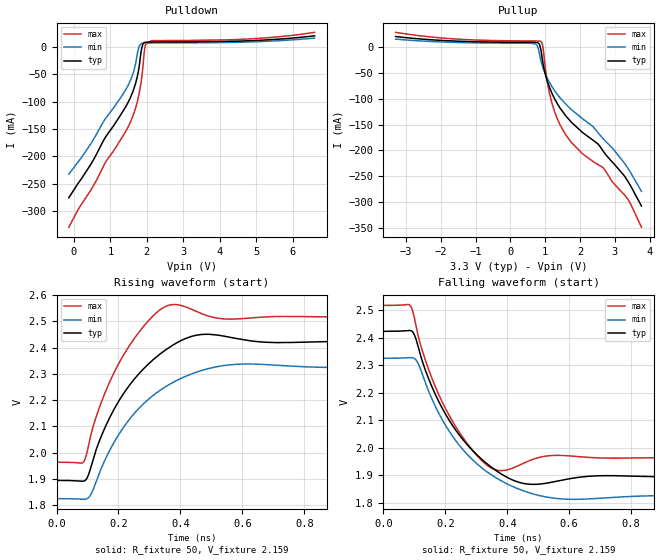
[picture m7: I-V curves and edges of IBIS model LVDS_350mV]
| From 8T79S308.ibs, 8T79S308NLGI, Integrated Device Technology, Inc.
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[Model]   LVDS_350mV
Model_type   Output
Polarity   Non-Inverting
|   typ   min   max
C_comp   2pF   1.5pF   2.5pF
Vmeas = 2.159V
Rref = 50
Cref = 0
Vref = 2.159V
|   typ   min   max
[Voltage range]   3.3V   3.135V   3.465V
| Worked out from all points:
|   slope of the pulldown table from 0 to 0.495 V, typ, clamps not added: 9.85 ohm
|   slope of the pullup table from 0 to 0.495 V, typ, clamps not added: 3.02 kohm
|   rising waveform, R_fixture 50, V_fixture 2.159: 20-80 % time 154ps typ, 180ps min, 122ps max; typ from 1.89 V to 2.42 V
|   falling waveform, R_fixture 50, V_fixture 2.159: 20-80 % time 154ps typ, 180ps min, 122ps max; typ from 2.42 V to 1.89 V
[Pulldown]
|Voltage   I (typ)   I (min)   I (max)
|Note, modeling breaks down at 250mA and above.  This is well beyond the functional   |
|operating range of the device.  Should this scenario occur, catastrophic failure and   |
|possible damage to the device and/or board is of higher concern than the I-V curve   |
|behavior.  The IBIS checker will flag currents in excess of 10A with warnings.  Lines   |
|with currents in excess of 0.35 A have been commented out.  The points still remain|
|available to the user if the user desires to use them.   |
|-1.60000e+00   -9.36050e-01   -8.30532e-01   -1.09194e+00
|-1.58360e+00   -9.23451e-01   -8.19980e-01   -1.07602e+00
|-1.51800e+00   -8.73064e-01   -7.77803e-01   -1.01237e+00
|-1.38680e+00   -7.72248e-01   -6.93503e-01   -8.84958e-01
|-1.32120e+00   -7.21791e-01   -6.51361e-01   -8.21228e-01
|-1.30480e+00   -7.09172e-01   -6.40828e-01   -8.05295e-01
|-1.27200e+00   -6.83929e-01   -6.19757e-01   -7.73430e-01
|-1.14080e+00   -5.82896e-01   -5.35437e-01   -6.46183e-01
|-1.07520e+00   -5.32359e-01   -4.93249e-01   -5.82891e-01
|-1.04240e+00   -5.07094e-01   -4.72151e-01   -5.51375e-01
|-9.76800e-01   -4.56591e-01   -4.29949e-01   -4.88499e-01
|-9.60400e-01   -4.43978e-01   -4.19400e-01   -4.73586e-01
|-9.27600e-01   -4.18775e-01   -3.98303e-01   -4.59203e-01
|-8.62000e-01   -3.73001e-01   -3.56137e-01   -4.46935e-01
|-7.96400e-01   -3.57891e-01   -3.14301e-01   -4.36605e-01
|-7.47200e-01   -3.51027e-01   -2.97867e-01   -4.28708e-01
|-6.81600e-01   -3.42516e-01   -2.88038e-01   -4.17953e-01
|-5.50400e-01   -3.25813e-01   -2.73543e-01   -3.96026e-01
|-5.34000e-01   -3.23742e-01   -2.71817e-01   -3.93266e-01
|-4.19200e-01   -3.09364e-01   -2.59932e-01   -3.73966e-01
|-4.02800e-01   -3.07325e-01   -2.58260e-01   -3.71225e-01
-140.4mV  -275.5mA   -232.5mA   -329.3mA
466.4mV   -214mA     -176.5mA   -261.2mA
860mV     -165.2mA   -131.3mA   -211.4mA
1.549V    -92.3mA    -61.1mA    -137.2mA
1.696V    -64.81mA   -28.55mA   -110.1mA
1.795V    -32.56mA   1.867mA    -82.65mA
1.877V    2.498mA    7.079mA    -45.82mA
1.926V    8.06mA     7.495mA    -10.52mA
1.959V    8.947mA    7.572mA    4.602mA
2.123V    9.35mA     7.638mA    11.84mA
4.73V     11.45mA    9.297mA    14.72mA
6.6V      20.66mA    16.55mA    27.05mA
[Pullup]
|Voltage   I (typ)   I (min)   I (max)
|Note, modeling breaks down at 250mA and above.  This is well beyond the functional   |
|operating range of the device.  Should this scenario occur, catastrophic failure and   |
|possible damage to the device and/or board is of higher concern than the I-V curve   |
|behavior.  The IBIS checker will flag currents in excess of 10A with warnings.  Lines   |
|with currents in excess of 0.35 A have been commented out.  The points still remain|
|available to the user if the user desires to use them.   |
-3.3V     20.66mA    15.57mA    28.83mA
719.4mV   9.383mA    6.524mA    12.05mA
798.6mV   8.199mA    -2.249mA   12mA
877.8mV   -5.663mA   -26.39mA   10.96mA
937.2mV   -31.68mA   -40.05mA   -604.3uA
1.016V    -55.6mA    -53.79mA   -47.49mA
1.115V    -76.39mA   -67.37mA   -86.96mA
1.432V    -118.4mA   -98.48mA   -151.1mA
2.066V    -164.9mA   -138.1mA   -206mA
2.68V     -202.6mA   -178.2mA   -234.6mA
3.373V    -259.2mA   -234.1mA   -294.4mA
3.769V    -307.8mA   -279.4mA   -348.7mA
| 3.84780e+00   -3.18622e-01   -2.89838e-01   -3.61401e-01
| 3.92700e+00   -3.29799e-01   -3.10228e-01   -3.74242e-01
| 3.96660e+00   -3.35470e-01   -3.35012e-01   -3.80702e-01
| 4.12500e+00   -3.60005e-01   -4.37435e-01   -4.06822e-01
| 4.16460e+00   -3.71679e-01   -4.63034e-01   -4.13410e-01
| 4.18440e+00   -3.83289e-01   -4.75832e-01   -4.16714e-01
| 4.22400e+00   -4.13932e-01   -5.01423e-01   -4.23349e-01
| 4.24380e+00   -4.29251e-01   -5.14216e-01   -4.26683e-01
| 4.40220e+00   -5.51718e-01   -6.16484e-01   -4.57199e-01
| 4.48140e+00   -6.12900e-01   -6.67560e-01   -5.22591e-01
| 4.50120e+00   -6.28190e-01   -6.80327e-01   -5.41875e-01
| 4.58040e+00   -6.89334e-01   -7.31378e-01   -6.18981e-01
| 4.89720e+00   -9.33601e-01   -9.36352e-01   -9.26929e-01
| 4.93680e+00   -9.64105e-01   -9.63467e-01   -9.65380e-01
| 4.95660e+00   -9.79356e-01   -9.77439e-01   -9.84604e-01
| 4.99620e+00   -1.00984e+00   -1.00618e+00   -1.02305e+00
| 5.07540e+00   -1.07073e+00   -1.06591e+00   -1.09992e+00
| 5.23380e+00   -1.19275e+00   -1.06591e+00   -1.25364e+00
| 5.31300e+00   -1.25569e+00   -1.06591e+00   -1.33049e+00
| 5.35260e+00   -1.28878e+00   -1.06591e+00   -1.36892e+00
| 5.51100e+00   -1.42874e+00   -1.06591e+00   -1.52275e+00
| 5.66940e+00   -1.42874e+00   -1.06591e+00   -1.67704e+00
| 5.76840e+00   -1.42874e+00   -1.06591e+00   -1.77893e+00
| 5.92680e+00   -1.42874e+00   -1.06591e+00   -1.95172e+00
| 5.94660e+00   -1.42874e+00   -1.06591e+00   -1.97363e+00
[Ramp]
|   typ   min   max
dV/dt_r   0.335/0.172n   0.309/0.191n   0.362/0.142n
dV/dt_f   0.335/0.172n   0.309/0.191n   0.362/0.142n
R_load =   50.0000
[Rising Waveform]
R_fixture = 50
V_fixture   =2.159  |Vcc_typ
V_fixture_min=2.075  |Vcc_min
V_fixture_max=2.220  |Vcc_max
C_fixture = 0.0p
| Time   typ   min   max
0s        1.894V     1.825V     1.964V
88.09ps   1.892V     1.822V     1.966V
110.1ps   1.941V     1.839V     2.064V
140.1ps   2.05V      1.928V     2.178V
204.2ps   2.203V     2.075V     2.347V
294.3ps   2.335V     2.201V     2.499V
366.4ps   2.403V     2.261V     2.563V
466.5ps   2.45V      2.312V     2.53V
594.6ps   2.432V     2.337V     2.51V
2ns       2.423V     2.325V     2.517V
[Falling Waveform]
R_fixture = 50
V_fixture   =2.159  |Vcc_typ
V_fixture_min=2.075  |Vcc_min
V_fixture_max=2.220  |Vcc_max
C_fixture = 0.0p
| Time   typ   min   max
0s        2.423V     2.325V     2.517V
88.09ps   2.426V     2.328V     2.515V
110.1ps   2.376V     2.311V     2.417V
140.1ps   2.268V     2.222V     2.303V
204.2ps   2.115V     2.075V     2.134V
294.3ps   1.982V     1.949V     1.982V
366.4ps   1.915V     1.889V     1.918V
466.5ps   1.868V     1.838V     1.951V
594.6ps   1.886V     1.813V     1.971V
2ns       1.894V     1.825V     1.964V
